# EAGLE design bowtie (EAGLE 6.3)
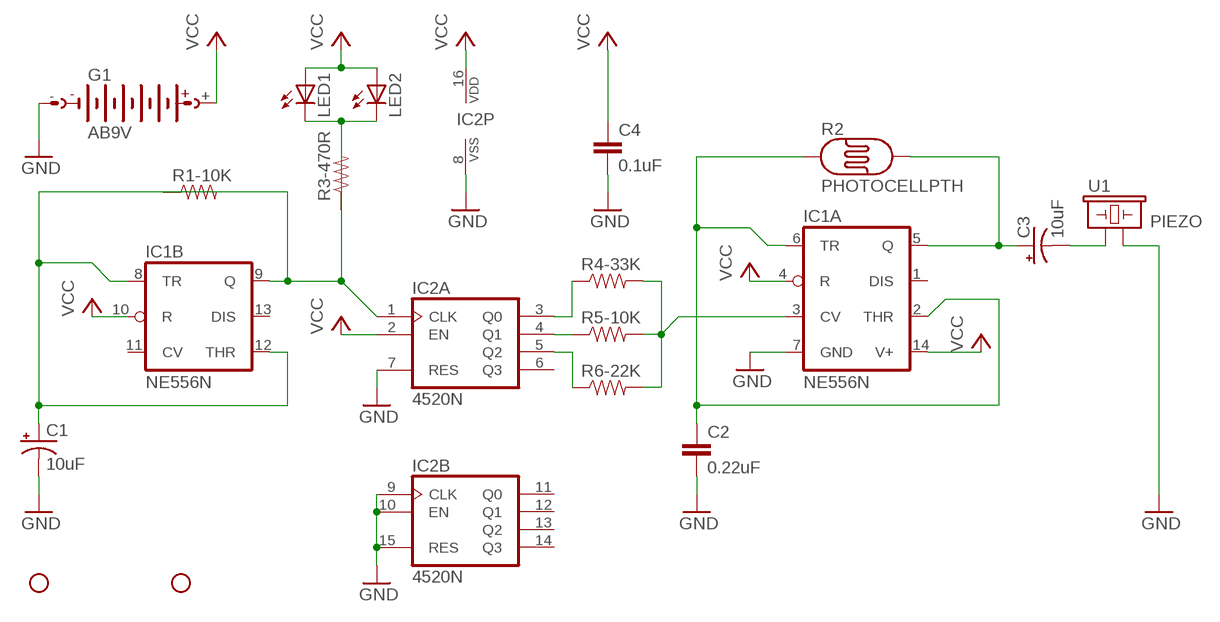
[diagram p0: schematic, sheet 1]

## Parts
C1  10uF  CAP_POLPTH1  [CPOL-RADIAL-100UF-25V]
C2  0.22uF  CAPPTH  [CAP-PTH-SMALL]
C3  10uF  CAP_POLPTH1  [CPOL-RADIAL-100UF-25V]
C4  0.1uF  CAPPTH  [CAP-PTH-SMALL]
G1  AB9V  [AB9V]
IC1  NE556N  [DIL14]
IC2  4520N  [DIL16]
LED1  LED10MM  [LED10MM]
LED2  LED10MM  [LED10MM]
R1-10K  RESISTORPTH-1/4W  [AXIAL-0.4]
R2  PHOTOCELLPTH  [PHOTOCELL]
R3-470R  RESISTORPTH-1/4W  [AXIAL-0.4]
R4-33K  RESISTORPTH-1/4W  [AXIAL-0.4]
R5-10K  RESISTORPTH-1/4W  [AXIAL-0.4]
R6-22K  RESISTORPTH-1/4W  [AXIAL-0.4]
STANDOFF1  STAND-OFF  [STAND-OFF]
STANDOFF2  STAND-OFF  [STAND-OFF]
U1  PIEZO  [PIEZO-12.6MM]

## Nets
GND: C1.2(-) C2.2 C4.2 G1.- IC1.7(A:GND) IC2.7(A:RES) IC2.8(P:VSS) IC2.9(B:CLK) IC2.10(B:EN) IC2.15(B:RES) U1.-
N$1: C3.1(+) IC1.5(A:Q) R2.2
N$2: C2.1 IC1.2(A:THR) IC1.6(A:TR) R2.1
N$3: IC1.9(B:Q) IC2.1(A:CLK) R1-10K.P$1 R3-470R.P$2
N$4: C1.1(+) IC1.8(B:TR) IC1.12(B:THR) R1-10K.P$2
N$5: LED1.K(C) LED2.K(C) R3-470R.P$1
N$6: IC2.3(A:Q0) R4-33K.P$1
N$7: C3.2(-) U1.+
N$8: IC2.4(A:Q1) R5-10K.P$1
N$9: IC2.5(A:Q2) R6-22K.P$1
N$10: IC1.3(A:CV) R4-33K.P$2 R5-10K.P$2 R6-22K.P$2
VCC: C4.1 G1.+ IC1.4(A:R) IC1.10(B:R) IC1.14(A:V+) IC2.2(A:EN) IC2.16(P:VDD) LED1.A LED2.A
Unconnected: IC1.1(A:DIS) IC1.11(B:CV) IC1.13(B:DIS) IC2.6(A:Q3) IC2.11(B:Q0) IC2.12(B:Q1) IC2.13(B:Q2) IC2.14(B:Q3)

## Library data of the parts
C1 C3 = SparkFun-Capacitors:CAP_POL: Capacitor Polarized
C2 C4 = SparkFun-Capacitors:CAP: Capacitor
G1 = battery:AB9V: 9-V BATTERY CLIP
IC1 = linear:*556: Dual TIMER
IC2 = big-mess-o-wires:4520: Dual binary up COUNTER
LED1 LED2 = led:LED: LED
R1-10K R3-470R R4-33K R5-10K R6-22K = SparkFun-Resistors:RESISTOR: Resistor
R2 = SparkFun-Sensors:PHOTOCELL: CdS photoresistor. This is a low cost way to detect light levels. Resistance decreases with more incoming light. SparkFun SKU: SEN-09088
STANDOFF1 STANDOFF2 = SparkFun-Electromechanical:STAND-OFF: #4 Stand Off
U1 = big-mess-o-wires:PIEZO: Piezo sounder

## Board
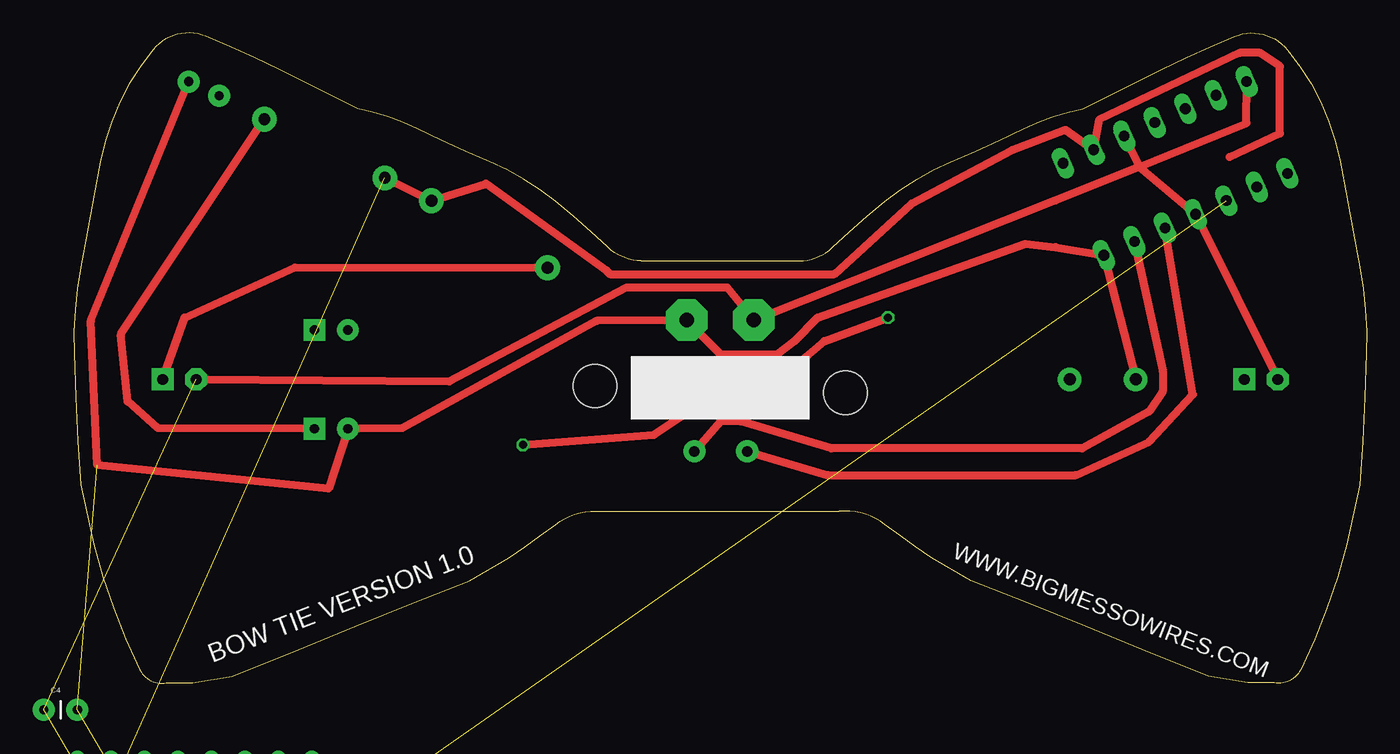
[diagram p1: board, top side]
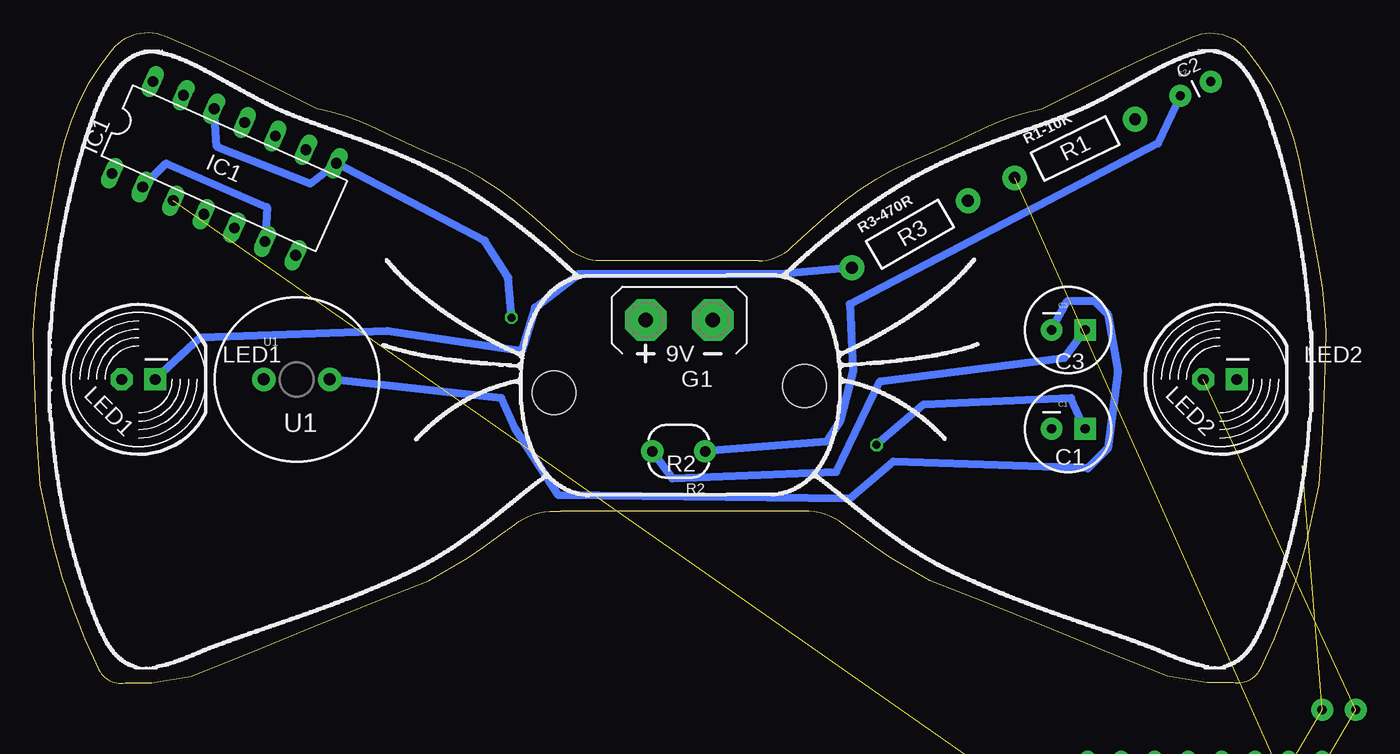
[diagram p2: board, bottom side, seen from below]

Size 98.01 x 49.29 mm. Coordinates in mm from the lower left corner, seen from the top.
Outline: 43,32.03 arc-44 40.5,33.03 arc5 36.5,36.53 arc16 31.5,39.53 arc-3 26,42.03 arc15 21.5,43.53 15.5,46.53 arc4 10,49.03 arc73 6,48.03 arc29 2,39.53 arc0 0.5,31.53 arc12 0,25.03 arc2 0.5,15.03 1.5,10.53 arc12 5,1.03 arc74 7,0.03 9,0.03 12,0.53 17,2.53 arc-2 30,7.78 33,9.53 arc4 36.5,12.03 arc-43 40,13.03 58,13.03 arc-43 61.5,12.03 arc4 65,9.53 68,7.78 arc-2 81,2.53 86,0.53 89,0.03 91,0.03 arc74 93,1.03 arc12 96.5,10.53 97.5,15.03 arc2 98,25.03 arc12 97.5,31.53 arc0 96,39.53 arc29 92,48.03 arc73 88,49.03 arc4 82.5,46.53 76.5,43.53 arc15 72,42.03 arc-3 66.5,39.53 arc16 61.5,36.53 arc5 57.5,33.03 arc-44 55,32.03 43,32.03
Copper layers (1*16): Top 0.0356mm / dielectric 1.5011mm / Bottom 0.0356mm
Design rules "LaenPCBOrder": minimum track width 6mil, minimum drill 13mil, track to track 6mil, track to pad 6mil, pad to pad 6mil, via to via 6mil, smd to smd 6mil, copper to edge 15mil, drill to drill 6mil, minimum pad ring 7mil, minimum via ring 7mil, stop-mask expansion 3mil, vias tented up to drill 0mil, thermal gap 10mil

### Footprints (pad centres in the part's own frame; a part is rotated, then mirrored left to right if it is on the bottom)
CPOL-RADIAL-100UF-25V = drill 0.7 pad 1.651 square: 1 1.27,0 | drill 0.7 pad 1.651: 2 -1.27,0
CAP-PTH-SMALL = drill 0.7 pad 1.651: 1 0,0; 2 2.54,0
AB9V = drill 1.118 pad 3.15 octagon: + 0,2.54; - 0,-2.54
DIL14 = drill 0.813 long: 1 -7.62,-3.81; 2 -5.08,-3.81; 3 -2.54,-3.81; 4 0,-3.81; 5 2.54,-3.81; 6 5.08,-3.81; 7 7.62,-3.81; 8 7.62,3.81; 9 5.08,3.81; 10 2.54,3.81; 11 0,3.81; 12 -2.54,3.81; 13 -5.08,3.81; 14 -7.62,3.81
DIL16 = drill 0.813 long: 1 -8.89,-3.81; 2 -6.35,-3.81; 3 -3.81,-3.81; 4 -1.27,-3.81; 5 1.27,-3.81; 6 3.81,-3.81; 7 6.35,-3.81; 8 8.89,-3.81; 9 8.89,3.81; 10 6.35,3.81; 11 3.81,3.81; 12 1.27,3.81; 13 -1.27,3.81; 14 -3.81,3.81; 15 -6.35,3.81; 16 -8.89,3.81
LED10MM = drill 0.813 pad 1.676 octagon: A -1.27,0 | drill 0.813 pad 1.676 square: K 1.27,0
AXIAL-0.4 = drill 0.9 pad 1.88: P$1 -5.08,0; P$2 5.08,0
PHOTOCELL = drill 0.8 pad 1.676: 1 -2,0; 2 2,0
STAND-OFF = hole 3.302: 0,0
PIEZO-12.6MM = drill 0.9 pad 1.778: + 2.5,0; - -2.5,0

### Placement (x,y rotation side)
C1  19.5,19.28 0 bottom
C2  11,44.53 25 bottom
C3  19.5,26.78 0 bottom
C4  -2.28,-2 0 top
G1  49,27.53 90 bottom
IC1  83.5,39.03 336 bottom
IC2  not placed on the board
LED1  90,23.03 0 bottom
LED2  8,23.03 0 bottom
R1-10K  19,40.53 26 bottom
R2  49.05,17.58 180 bottom
R3-470R  31.5,34.03 30 bottom
R4-33K  not placed on the board
R5-10K  not placed on the board
R6-22K  not placed on the board
STANDOFF1  39.5,22.53 0 top
STANDOFF2  58.5,22.03 0 top
U1  78,23.03 0 bottom

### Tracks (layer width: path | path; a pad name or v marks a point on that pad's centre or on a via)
GND  (6 unrouted)
  Top 0.61: U1.- IC1.7 74.43,33.05 72.14,33.3 56.39,27.72 54.61,25.94 53.34,24.92 49.03,24.92 G1.- 39.63,27.46 24.9,19.33 C1.2 19.31,14.76 1.78,16.54 1.27,27.46 C2.2
N$1
  Top 0.61: R2.2 57.15,15.78 75.95,15.78 81.54,18.32 84.84,21.87 IC1.5
  Bottom 0.61: R2.2 49.53,15.52 37.09,16.03 33.79,22.89 19.82,24.67 C3.1
N$2
  Top 0.61: IC1.6 82.55,23.65 82.55,22.13 81.54,20.6 76.46,17.81 57.41,17.81 50.55,19.84 49.03,19.84 R2.1
  Bottom 0.61: IC1.2 87.89,39.4 80.27,36.1 IC1.6 | C2.1 12.7,40.92 36.07,28.73 35.82,23.65 36.83,19.84 37.85,18.32 R2.1
N$3  (1 unrouted)
  Top 0.61: 87.63,39.91 91.44,41.69 91.44,46.77 89.92,47.78 88.4,47.78 77.73,42.7 IC1.9 75.19,41.94 71.12,40.42 63.5,36.35 57.66,31.02 40.64,31.02 40.39,31.27 31.25,37.88 R3-470R.P$2 R1-10K.P$1
N$4  (via drill 0.6)
  Top 0.61: C1.1 6.35,19.33 4.07,21.37 3.56,26.45 R1-10K.P$2 | v34.04,18.06 43.95,18.83 49.28,22.38 53.6,23.14 56.9,25.94 v61.73,27.72
  Bottom 0.61: IC1.12 84.08,40.67 76.97,37.88 IC1.8 63.76,33.56 61.98,30.76 v61.73,27.72 | C1.1 19.31,21.62 30.48,21.11 v34.04,18.06
N$5
  Top 0.61: LED2.K 8.39,27.72 16.77,31.53 R3-470R.P$1
  Bottom 0.61: R3-470R.P$1 41.41,31.02 56.65,31.02 59.95,28.48 60.96,25.18 71.12,26.7 85.35,26.19 LED1.K
N$6  (1 unrouted)
N$7
  Bottom 0.61: C3.2 19.56,28.99 17.53,28.99 16.51,27.97 15.75,23.65 16.51,17.81 18.04,16.29 32.77,16.79 36.07,14 58.17,14.25 61.47,19.33 62.49,21.62 U1.+
N$8  (1 unrouted)
N$9  (1 unrouted)
N$10  (3 unrouted)
VCC  (3 unrouted)
  Top 0.61: 80.78,39.15 74.43,36.61 G1.+ 49.53,30 41.91,30 28.45,22.89 LED2.A | 80.78,39.15 IC1.4 LED1.A | IC1.10 80.78,39.15 | 80.78,39.15 88.9,42.45 IC1.14

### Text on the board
tPlace: WWW.BIGMESSOWIRES.COM | BOW TIE VERSION 1.0
bPlace: C2 | R1 | IC1 | R3 | _ | _ | C3 | LED2 | LED1 | U1 | C1 | R2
